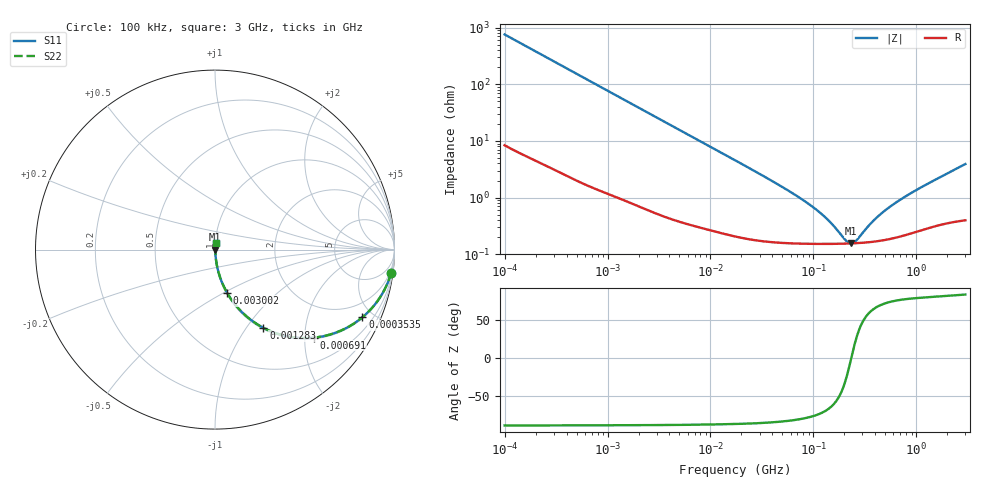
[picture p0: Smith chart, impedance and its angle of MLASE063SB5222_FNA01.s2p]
! MLASE063SB5222_FNA01  S-PARAMETER MODEL  ( Standard Model )
! Model Generated by TAIYO YUDEN Corporation (http://www.ty-top.com)
! Version 1.0
! TAIYO YUDEN Control No. 220601
! Copyright(c) 2007 TAIYO YUDEN CO.,LTD. All Rights Reserved.
! Product Description (link to TY-COMPAS)
! https://ds.yuden.co.jp/TYCOMPAS/or/detail?pn=MLASE063SB5222KFNA01&u=M
! Products Name : Multilayer Ceramic Capacitors
! Characteristics :
!  Capacitance : 2200 [pF] , Rated Voltage : 16 [V] , TCC : B / X5R
!  Case Size : 0.6 x 0.3 / 0.024 x 0.012 [mm/inch] , Thickness : 0.3 / 0.012 [mm/inch]
!  (Conditions: Temperature = 25 [degC] , DC Bias Voltage = 0 [V])
! External Node Assignments :
!  1  o---| |---o  2
! GND o---------o GND
! Frequency Range : 100kHz  -  3GHz  [ 401 STEP ]
# MHZ S RI R 50
! Freq[MHz].  S11 Real  S11 Imag  S21 Real  S21 Imag  S12 Real  S12 Imag  S22 Real  S22 Imag
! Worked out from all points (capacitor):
!   401 points, 100 kHz to 3 GHz, reference 50 ohm
!   read as one part in series: C = 2.09 nF near 105.3 kHz
!   lowest |Z| = 155 mohm at 233.9 MHz (marker M1)
!   series resonance near 233.5 MHz, so ESL is about 220 pH
!   S11 on the Smith chart (normalised r, x): 100 kHz: 1, -15; 353.5 kHz: 1.05, -4.33; 691 kHz: 1.03, -2.23; 1.283 MHz: 1.02, -1.21; 3.002 MHz: 1.01, -0.52; 3 GHz: 1.01, +0.08
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0.1  0.9816 -0.129  0.0184 0.129  0.0184 0.129  0.9816 -0.129
0.205778  0.9296 -0.2499  0.0704 0.2499  0.0704 0.2499  0.9296 -0.2499
0.353547  0.8213 -0.3769  0.1787 0.3769  0.1787 0.3769  0.8213 -0.3769
0.562235  0.6495 -0.4706  0.3505 0.4706  0.3505 0.4706  0.6495 -0.4706
0.690972  0.553 -0.4904  0.447 0.4904  0.447 0.4904  0.553 -0.4904
0.917447  0.4153 -0.4855  0.5847 0.4855  0.5847 0.4855  0.4153 -0.4855
1.282589  0.2701 -0.436  0.7299 0.436  0.7299 0.436  0.2701 -0.436
1.937191  0.1429 -0.3412  0.8571 0.3412  0.8571 0.3412  0.1429 -0.3412
3.002272  0.0674 -0.241  0.9326 0.241  0.9326 0.241  0.0674 -0.241
3.161081  0.0616 -0.2305  0.9384 0.2305  0.9384 0.2305  0.0616 -0.2305
6.848882  0.016 -0.1125  0.984 0.1125  0.984 0.1125  0.016 -0.1125
17.7727  0.00399 -0.0442  0.996 0.0442  0.996 0.0442  0.00399 -0.0442
52.46276  0.00178 -0.0144  0.9982 0.0144  0.9982 0.0144  0.00178 -0.0144
97.38194  0.00156 -0.00677  0.9984 0.00677  0.9984 0.00677  0.00156 -0.00677
139.694  0.00153 -0.00367  0.9985 0.00367  0.9985 0.00367  0.00153 -0.00367
205.6221  0.00153 -0.00087  0.9985 0.00087  0.9985 0.00087  0.00153 -0.00087
233.9019  0.00155 1.29e-05  0.9985 -1.29e-05  0.9985 -1.29e-05  0.00155 1.29e-05
259.3015  0.00156 0.000718  0.9984 -0.000718  0.9984 -0.000718  0.00156 0.000718
381.6779  0.00167 0.00348  0.9983 -0.00348  0.9983 -0.00348  0.00167 0.00348
547.5153  0.00188 0.00648  0.9981 -0.00648  0.9981 -0.00648  0.00188 0.00648
1016.304  0.00267 0.0135  0.9973 -0.0135  0.9973 -0.0135  0.00267 0.0135
3000  0.00544 0.0386  0.9946 -0.0386  0.9946 -0.0386  0.00544 0.0386
